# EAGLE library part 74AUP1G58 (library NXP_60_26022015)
Low-power configurable multiple function gate The 74AUP1G58 provides configurable multiple functions. The output state is determined by eight patterns of 3-bit input. The user can choose the logic functions AND, OR, NAND, NOR, XOR, inverter and buffer. All inputs can be connected to VCC or GND. This device ensures a very low static and dynamic power consumption across the entire VCC range from 0.8 V to 3.6 V. This device is fully specified for partial power-down applications using IOFF. The IOFF circuitry disables the output, preventing the damaging backflow current through the device when it is powered down. The 74AUP1G58 has Schmitt trigger inputs making it capable of transforming slowly changing input signals into sharply defined, jitter-free output signals. The inputs switch at different points for positive and negative-going signals. The difference between the positive voltage VT+ and the negative voltage VT- is defined as the input hysteresis voltage VH. AAL Eindhoven MK
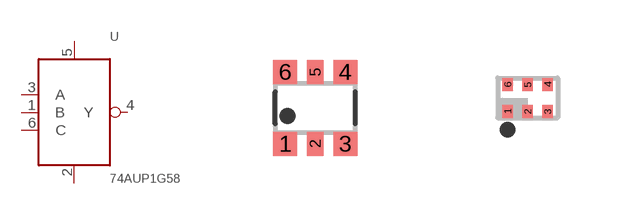
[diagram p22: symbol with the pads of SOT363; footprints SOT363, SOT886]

Designator prefix U

## 74AUP1G58GW (12NC: 9352 799 59125)  [SOT363]
1  B  in
2  GND  pwr
3  A  in
4  Y  out
5  VCC  pwr
6  C  in

## 74AUP1G58GM (12NC: 9352 799 61132)  [SOT886]
Pads as for SOT363

## 74AUP1G58GF (12NC: 9352 813 29132)  [SOT891]
Pads as for SOT363

## 74AUP1G58GS (12NC: 9352 928 68132)  [SOT1202]
Pads as for SOT363

## 74AUP1G58GN (I2C: 9352 917 44132)  [SOT1115]
Pads as for SOT363

## Footprint SOT363 (pad centres in mm)
SOT363 Plastic surface-mounted package; 6 leads JEDEC: -- IEC: -- JEITA: SC-88
smd 0.6 x 0.6: 1 -0.75,-0.9; 3 0.75,-0.9; 4 0.75,0.9; 6 -0.75,0.9
smd 0.4 x 0.6: 2 0,-0.9; 5 0,0.9

## Footprint SOT886 (pad centres in mm)
SOT886 XSON6: plastic extremely thin small outline package; no leads; 6 terminals; body 1 x 1.45 x 0.5 mm JEDEC: MO-252 IEC: ---
smd 0.27 x 0.325: 1 -0.5,-0.338; 2 0,-0.338; 3 0.5,-0.338; 4 0.5,0.338; 5 0,0.338; 6 -0.5,0.338

## Footprint SOT891 (pad centres in mm)
SOT891 XSON6: plastic extremely thin small outline package; no leads; 6 terminals; body 1 x 1 x 0.5 mm JEDEC: -- IEC: ---
smd 0.15 x 0.5: 1 -0.35,-0.35; 2 0,-0.35; 3 0.35,-0.35; 4 0.35,0.35; 5 0,0.35; 6 -0.35,0.35

## Footprint SOT1202 (pad centres in mm)
SOT1202 XSON6: extremely thin small outline package; no leads; 6 terminals; body 1.0 x 1.0 x 0.35 mm JEDEC: --- IEC: ---
smd 0.15 x 0.5: 1 -0.35,-0.35; 2 0,-0.35; 3 0.35,-0.35; 4 0.35,0.35; 5 0,0.35; 6 -0.35,0.35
